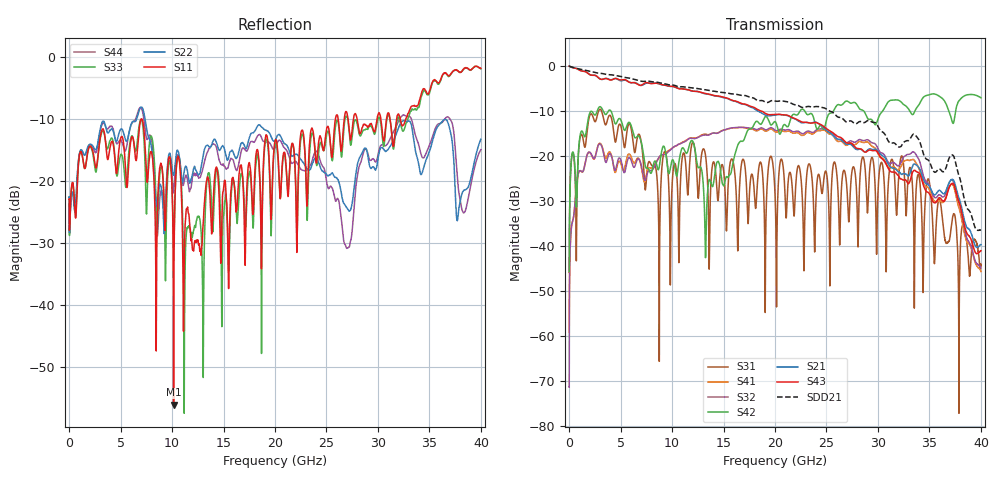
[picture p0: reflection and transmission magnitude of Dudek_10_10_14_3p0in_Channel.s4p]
! Created Thu Oct 09 16:28:00 2014
# hz S ma R 50
! 4 Port Network Data from SP1.SP block
! freq  magS11  angS11  magS12  angS12  magS13  angS13  magS14  angS14
!  magS21  angS21  magS22  angS22  magS23  angS23  magS24  angS24
!  magS31  angS31  magS32  angS32  magS33  angS33  magS34  angS34
!  magS41  angS41  magS42  angS42  magS43  angS43  magS44  angS44
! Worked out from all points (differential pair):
!   4001 points, 10 kHz to 40 GHz, reference 50 ohm
!   strongest paths, dB at 10 kHz, 10 GHz, 20 GHz, 30 GHz, 40 GHz:
!     S43: -0.1, -4.6, -10.8, -19.3, -41.1
!     S21: -0.1, -4.6, -11.0, -19.0, -39.7
!     S42: -45.7, -21.0, -12.4, -11.8, -7.1
!     S32: -71.3, -18.4, -14.3, -18.4, -44.9
!     S41: -59.1, -18.3, -14.6, -19.5, -45.7
!     S31: -45.9, -26.6, -28.4, -28.3, -44.1
!   taken as a pair (ports 3,1 in; 4,2 out), SDD21 dB: -0.1, -4.3, -7.8, -13.5, -36.6
!   lowest |S11| = -56.0 dB at 10.15 GHz (marker M1), VSWR 1.00, Z = 49.9 + j0.118 ohm
!   |S11| at or under -10 dB: start of sweep to 25.87 GHz; 27.97 GHz to 29.92 GHz (1.947 GHz wide, 6.73 % of centre); 31.17 GHz to 31.81 GHz (640.5 MHz wide, 2.03 % of centre)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
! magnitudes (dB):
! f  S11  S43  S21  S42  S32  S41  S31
! 10 kHz  -23.0  -0.1  -0.1  -45.7  -71.3  -59.1  -45.9
! 310 MHz  -20.3  -0.4  -0.4  -19.4  -34.8  -34.7  -19.5
! 1.83 GHz  -15.2  -1.7  -1.7  -12.1  -19.4  -19.4  -12.9
! 10.15 GHz  -56.0  -4.6  -4.7  -21.2  -18.1  -18.0  -22.4
! 27.06 GHz  -9.7  -17.2  -17.5  -7.9  -17.0  -17.6  -30.2
! 33.48 GHz  -7.9  -23.3  -21.8  -10.6  -19.1  -20.8  -36.5
! 40 GHz  -1.9  -41.1  -39.7  -7.1  -44.9  -45.7  -44.1
